(* Logix 5000 AddOnInstructionDefinition export Banner_LE_Param_v4; software revision 33.00 *)

TYPE Banner_IOL_Port_v4 :   // UDT that has all of the data items necessary to communicate with a specific Port on a IO-Link Master
STRUCT
   Port_Controlled : INT;   // Each bit represents a port on an IO-Link Master. Set to 1 to tell AOI to control that port.
   Port_Activate : INT;   // Each bit represents a port on an IO-Link Master. When ON that port will process any commands in queue.
   Port_Read : INT;   // Each bit represents a port on an IO-Link Master. Used to determine when device AOI has requested a Read command.
   Port_Write : INT;   // Each bit represents a port on an IO-Link Master. Used to determine when device AOI has requested a Write command.
   Port_RW_Complete : INT;   // Each bit represents a port on an IO-Link Master. Tells device AOI that Read or Write request has been completed.
   Port_Device_Read : INT;
   Data_Transfer : SINT[190];   // Array to transfer data from IO-Master to device AOIs.
END_STRUCT
END_TYPE

TYPE Banner_LE_RD_v4 :   // UDT with all of the Read only parameters for LE.
STRUCT
   Master_Cycle_Time : INT;
   Min_Cycle_Time : INT;
   M_Sequence_Capability : INT;
   IO_Link_Version_ID : INT;
   Process_Data_Input_Length : INT;
   Process_Data_Output_Length : INT;
   Combined_Vendor_ID : DINT;   // IO-Link Vendor ID
   Vendor_ID1 : INT;
   Vendor_ID2 : INT;
   Combined_Device_ID : DINT;   // IO-Link Device ID
   Device_ID1 : INT;
   Device_ID2 : INT;
   Device_ID3 : INT;
   Serial_Number : STRING;
   Teach_State : SINT;   // 0 =IDLE, 1 = SP1 Success, 4 = Wait for Command, 5 = Busy, 7 = Error
   SP1_TP1 : SINT;   // 0 = not taught or unsuccessful, 1 = successfully taught
   SP2_TP2 : SINT;   // 0 = not taught or unsuccessful, 1 = successfully taught
   Measurement_Value : DINT;   // Measurement value in .1 mm.
   Excess_Gain_Percent : DINT;   // Excess gain expressed as a percentage of minimum signal.
   Stability : INT;   // 0 = No target exists, 1 = Marginal or multiple peaks, 2 = Stable
   Laser_Fault_Status : DINT;   // 0 = No fault, 1 = Laser shut down due to a fault.
   Display_String : STRING;   // String currently being displayed on the LED display of the sensor
END_STRUCT
END_TYPE

TYPE Banner_LE_v4 :   // UDT with all of the parameters for LE.
STRUCT
   Initial_Global_Read : BOOL;   // Determines if all of the IO-Link data has been read into the PLC yet
   Command : INT;   // Value placed in here will activate a read or write to a specifc IO-Link Index
   Read_Data : Banner_LE_RD_v4;   // All read data
   Write_Data : Banner_LE_WD_v4;   // All data that can be written to.
   Archive : Banner_LE_WD_v4;   // Archive of the write data.
   Reset : BOOL;
END_STRUCT
END_TYPE

TYPE Banner_LE_WD_v4 :   // UDT that stores the Write Data for a LE.
STRUCT
   System_Command : INT;   // See IODD file for list of commands that can be activated via the System Command interface
   Parameter_Access_Lock : SINT;   // Write access to all read/write parameters is block when this bit is ON.
   Data_Storage_Lock : SINT;   // Data storage mechanism is inhibited when bit is ON.
   Local_Parameterization_Lock : SINT;   // Parameteriation via local control elementes is inhibited.
   Local_User_Interface_Lock : SINT;   // Operation of the hmi on the device is disabled.
   Teach_Channel : INT;   // 0 = Default, 1 = BDC1, 2 = BDC2
   BDC1_Setpoint_SP1 : DINT;   // SP1 switch point in Switch or Window mode. LE250: Range 100 to 400 (.1 mm increments). LE550: Range 100 to 1000 (.1 mm increments).
   BDC1_Setpoint_SP2 : DINT;   // SP1 switch point in Switch or Window mode. LE250: Range 100 to 400 (.1 mm increments). LE550: Range 100 to 1000 (.1 mm increments).
   BDC1_Swithpoint_Logic : INT;   // Discrete output only. 0 = Light Operate, 1 = Dark Operate
   BDC1_BDC_Mode : INT;   // 1 = Switch Mode/Single Point Mode, 2 = Window Mode, 132 = Health(LO)/Alarm Mode(DO)
   BDC1_Hysteresis : DINT;   // Not Used
   BDC2_Setpoint_SP1 : DINT;   // SP1 switch point in Switch or Window mode. LE250: Range 100 to 400 (.1 mm increments). LE550: Range 100 to 1000 (.1 mm increments).
   BDC2_Setpoint_SP2 : DINT;   // SP1 switch point in Switch or Window mode. LE250: Range 100 to 400 (.1 mm increments). LE550: Range 100 to 1000 (.1 mm increments).
   BDC2_Switchpoint_Logic : INT;   // Discrete output only. 0 = Light Operate, 1 = Dark Operate
   BDC2_BDC_Mode : INT;   // 1 = Switch Mode/Single Point Mode, 2 = Window Mode, 132 = Health(LO)/Alarm Mode(DO)
   BDC2_Hysteresis : DINT;   // Not Used
   Response_Speed : INT;   // 0 = Fast, 1 = Standard, 2 = Medium, 3 = Slow
   Zero_Reference_Location : INT;   // 0 = Near, 1 = Far
   Shift_Zero_Reference_After_Teach : INT;   // 0 = Off, 1 = AutoSet, 2 = SetZero
   Sensor_Lockout : SINT;   // 0 = No Lock Out, 1 = Sensor Locked
   IOL_Filter_Time : DINT;   // Time to average IOL process data measurement between updates. 0 to 65535 ms.
   Display_Read : SINT;   // 0 = Nomral, 1 = Inverted
   Display_Units : SINT;   // 0 = mm, 1 = inches
   Display_Sleep : SINT;   // 0 = 1 min, 1 = 5 min, 2 = 15 min, 3 = 60 min, 4 = Disabled
   Remote_Input_Type : SINT;   // 0 = Teach, 1 = Laser Enable, 2 = Sync Master, 3 = Sync Slave, 4 = Disabled
   BDC1_Delay_Mode : INT;   // 0 = Delay timer disabled, 1 = On & Off Delay, 2 = Off One-Shot timer, 3 = On One-Shot timer
   BDC1_Delay_On_OneShot_Delay : DINT;   // 0 to 9999 ms. 0 ms disables On delay or On/Off oneshot delay.
   BDC1_Delay_Off_OneShot_Delay : DINT;   // 0 to 9999 ms. 0 ms disables Off delay or On/Off oneshot delay.
   BDC1_Switch_Point_Reference : INT;   // 0 = Object, 1 = Background, 2 = Custom
   BDC1_User_Teach_Offset : DINT;   // Range 0 to 32767 (0 to 3276.7 mm)
   BDC1_Midpoint_Window_Size : DINT;   // Range 0 to 32767 (0 to 3276.7 mm)
   BDC1_Midpoint_Teach_Offset_Size : DINT;   // Range 0 to 32767 (0 to 3276.7 mm)
   BDC2_Delay_Mode : INT;   // 0 = Delay timer disabled, 1 = On & Off Delay, 2 = Off One-Shot timer, 3 = On One-Shot timer
   BDC2_Delay_On_OneShot_Delay : DINT;   // 0 to 9999. 0 ms disables On delay or On/Off oneshot delay.
   BDC2_Delay_Off_OneShot_Delay : DINT;   // 0 to 9999. 0 ms disables Off delay or On/Off oneshot delay.
   BDC2_Switch_Point_Reference : INT;   // 0 = Object, 1 = Background, 2 = Custom
   BDC2_User_Teach_Offset : DINT;   // Range 0 to 32767 (0 to 3276.7 mm)
   BDC2_Midpoint_Window_Size : DINT;   // Range 0 to 32767 (0 to 3276.7 mm)
   BDC2_Midpoint_Teach_Offset_Size : DINT;   // Range 0 to 32767 (0 to 3276.7 mm)
END_STRUCT
END_TYPE

ADD_ON_INSTRUCTION Banner_LE_Param_v4   (* revision 4.0, vendor Banner Engineering *)
// AOI to read and write parameter data to an IO-Link LE.
VAR_IN_OUT
   LE : Banner_LE_v4; {required}
   Port_Data : Banner_IOL_Port_v4; {required}
END_VAR
VAR_INPUT
   Port : DINT; {required}
END_VAR
VAR
   Local_Control : DINT; {access None}
   Global_Read_Command_Value : INT; {access None}
   Global_Write_Command_Value : INT; {access None}
   Command_Being_Processed : BOOL; {access None}
   Update_Archive : BOOL; {access None}
   Index_Write_Control : DINT; {access None}
   Index_Write_Inprocess : INT; {access None}
   Temp_Excess_Gain : DINT[2]; {access None}
   Inprocess_Index : DINT; {access None}
END_VAR

ROUTINE Logic   (* ladder *)
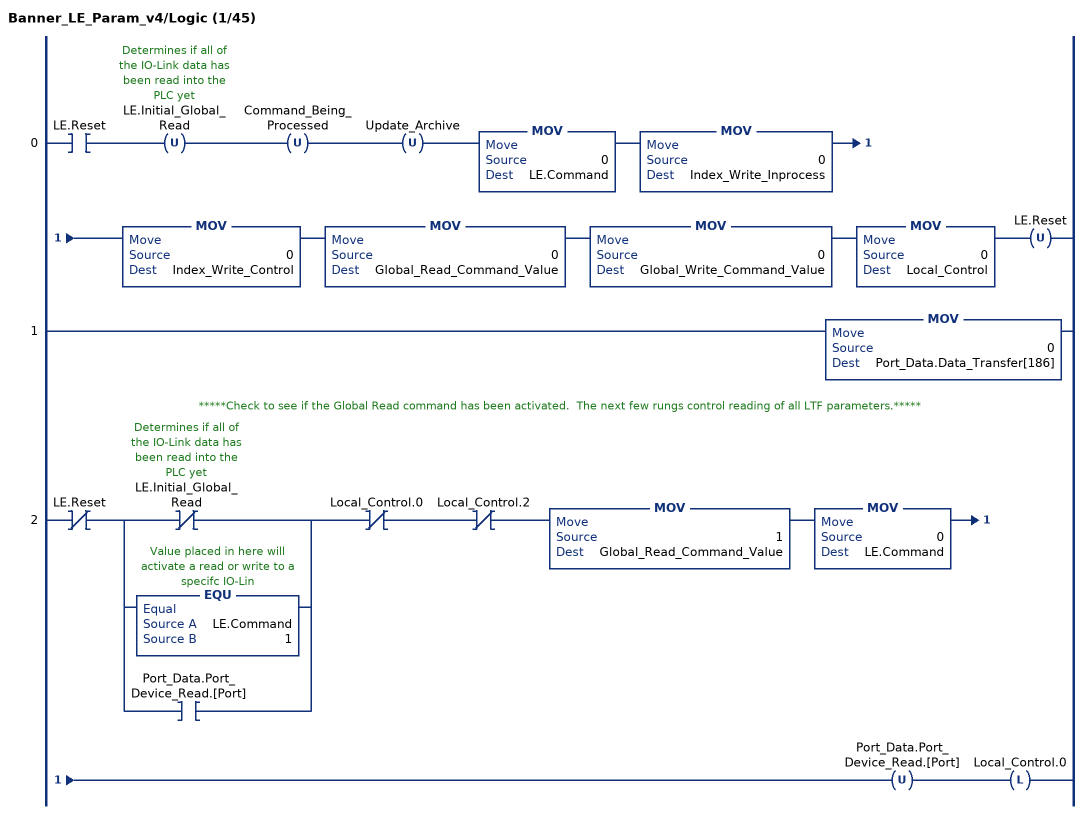
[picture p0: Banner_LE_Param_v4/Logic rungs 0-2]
   0: XIC(LE.Reset)OTU(LE.Initial_Global_Read)OTU(Command_Being_Processed)OTU(Update_Archive)MOV(0,LE.Command)MOV(0,Index_Write_Inprocess)MOV(0,Index_Write_Control)MOV(0,Global_Read_Command_Value)MOV(0,Global_Write_Command_Value)MOV(0,Local_Control)OTU(LE.Reset);
   1: MOV(0,Port_Data.Data_Transfer[186]);
   // *****Check to see if the Global Read command has been activated.  The next few rungs control reading of all LTF parameters.*****
   2: XIO(LE.Reset)[XIO(LE.Initial_Global_Read) ,EQU(LE.Command,1) ,XIC(Port_Data.Port_Device_Read.[Port]) ]XIO(Local_Control.0)XIO(Local_Control.2)MOV(1,Global_Read_Command_Value)MOV(0,LE.Command)OTU(Port_Data.Port_Device_Read.[Port])OTL(Local_Control.0);
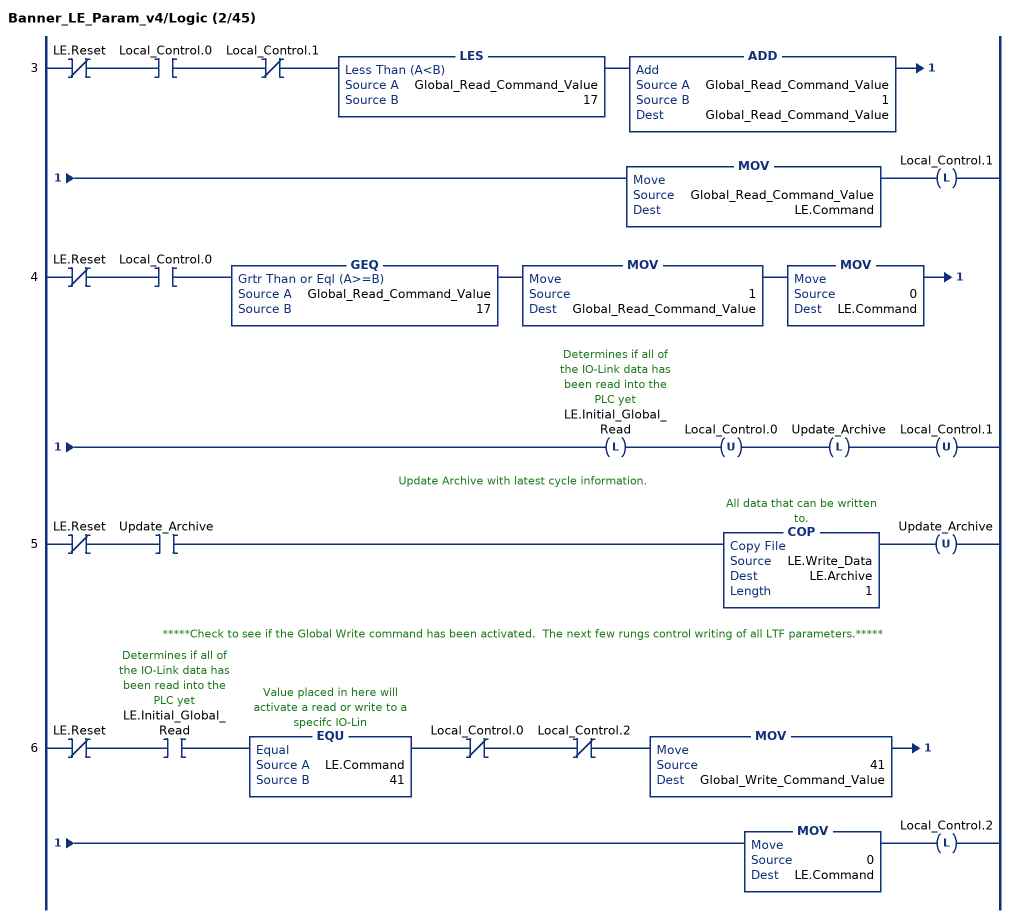
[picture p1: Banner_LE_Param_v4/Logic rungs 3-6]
   3: XIO(LE.Reset)XIC(Local_Control.0)XIO(Local_Control.1)LES(Global_Read_Command_Value,17)ADD(Global_Read_Command_Value,1,Global_Read_Command_Value)MOV(Global_Read_Command_Value,LE.Command)OTL(Local_Control.1);
   4: XIO(LE.Reset)XIC(Local_Control.0)GEQ(Global_Read_Command_Value,17)MOV(1,Global_Read_Command_Value)MOV(0,LE.Command)OTL(LE.Initial_Global_Read)OTU(Local_Control.0)OTL(Update_Archive)OTU(Local_Control.1);
   // Update Archive with latest cycle information.
   5: XIO(LE.Reset)XIC(Update_Archive)COP(LE.Write_Data,LE.Archive,1)OTU(Update_Archive);
   // *****Check to see if the Global Write command has been activated.  The next few rungs control writing of all LTF parameters.*****
   6: XIO(LE.Reset)XIC(LE.Initial_Global_Read)EQU(LE.Command,41)XIO(Local_Control.0)XIO(Local_Control.2)MOV(41,Global_Write_Command_Value)MOV(0,LE.Command)OTL(Local_Control.2);
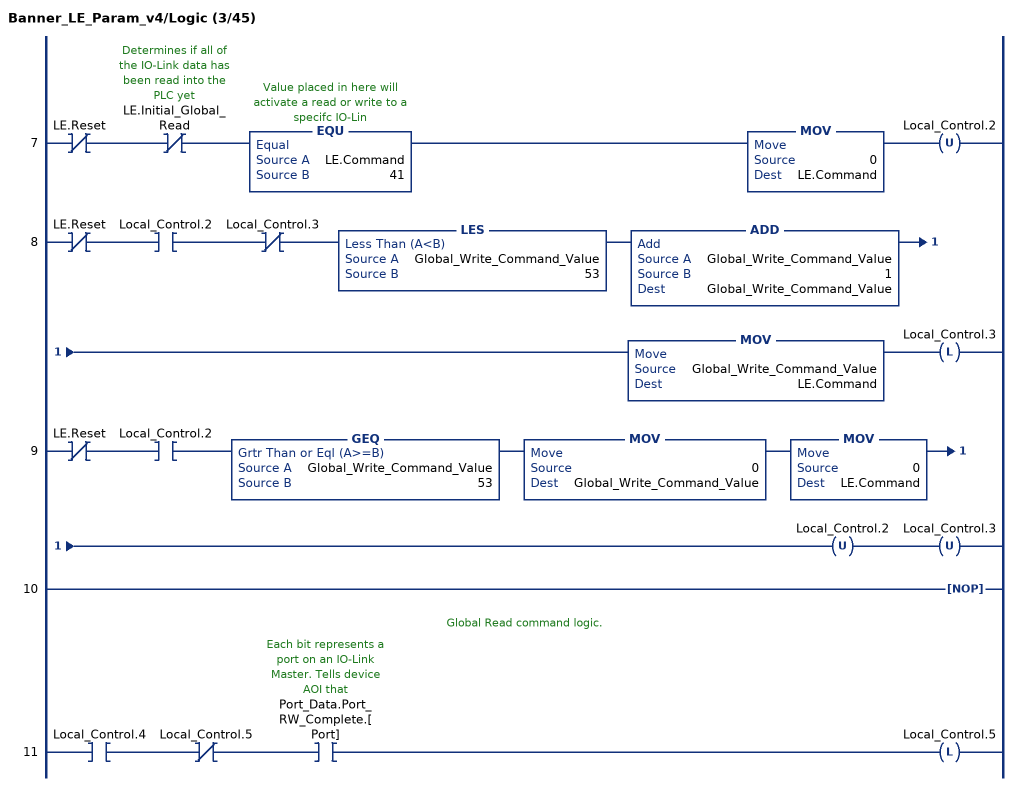
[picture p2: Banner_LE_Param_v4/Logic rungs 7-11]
   7: XIO(LE.Reset)XIO(LE.Initial_Global_Read)EQU(LE.Command,41)MOV(0,LE.Command)OTU(Local_Control.2);
   8: XIO(LE.Reset)XIC(Local_Control.2)XIO(Local_Control.3)LES(Global_Write_Command_Value,53)ADD(Global_Write_Command_Value,1,Global_Write_Command_Value)MOV(Global_Write_Command_Value,LE.Command)OTL(Local_Control.3);
   9: XIO(LE.Reset)XIC(Local_Control.2)GEQ(Global_Write_Command_Value,53)MOV(0,Global_Write_Command_Value)MOV(0,LE.Command)OTU(Local_Control.2)OTU(Local_Control.3);
   10: NOP();
   // Global Read command logic.
   11: XIC(Local_Control.4)XIO(Local_Control.5)XIC(Port_Data.Port_RW_Complete.[Port])OTL(Local_Control.5);
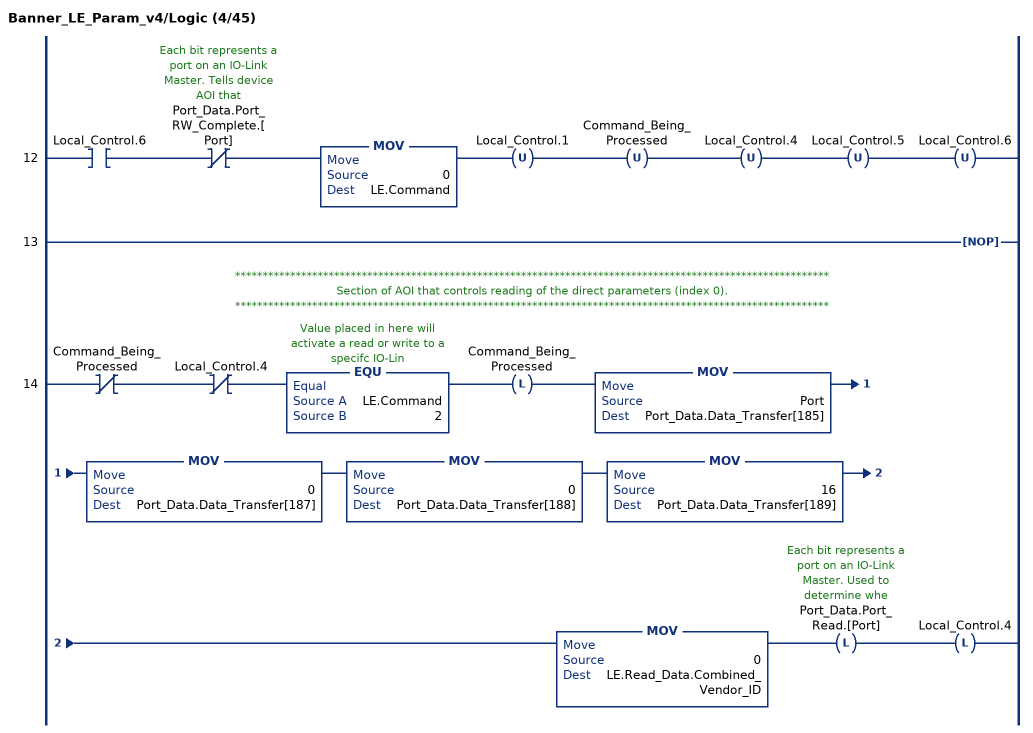
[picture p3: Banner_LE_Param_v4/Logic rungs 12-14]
   12: XIC(Local_Control.6)XIO(Port_Data.Port_RW_Complete.[Port])MOV(0,LE.Command)OTU(Local_Control.1)OTU(Command_Being_Processed)OTU(Local_Control.4)OTU(Local_Control.5)OTU(Local_Control.6);
   13: NOP();
   // ************************************************************************************************************
   // Section of AOI that controls reading of the direct parameters (index 0).
   // ************************************************************************************************************
   14: XIO(Command_Being_Processed)XIO(Local_Control.4)EQU(LE.Command,2)OTL(Command_Being_Processed)MOV(Port,Port_Data.Data_Transfer[185])MOV(0,Port_Data.Data_Transfer[187])MOV(0,Port_Data.Data_Transfer[188])MOV(16,Port_Data.Data_Transfer[189])MOV(0,LE.Read_Data.Combined_Vendor_ID)OTL(Port_Data.Port_Read.[Port])OTL(Local_Control.4);
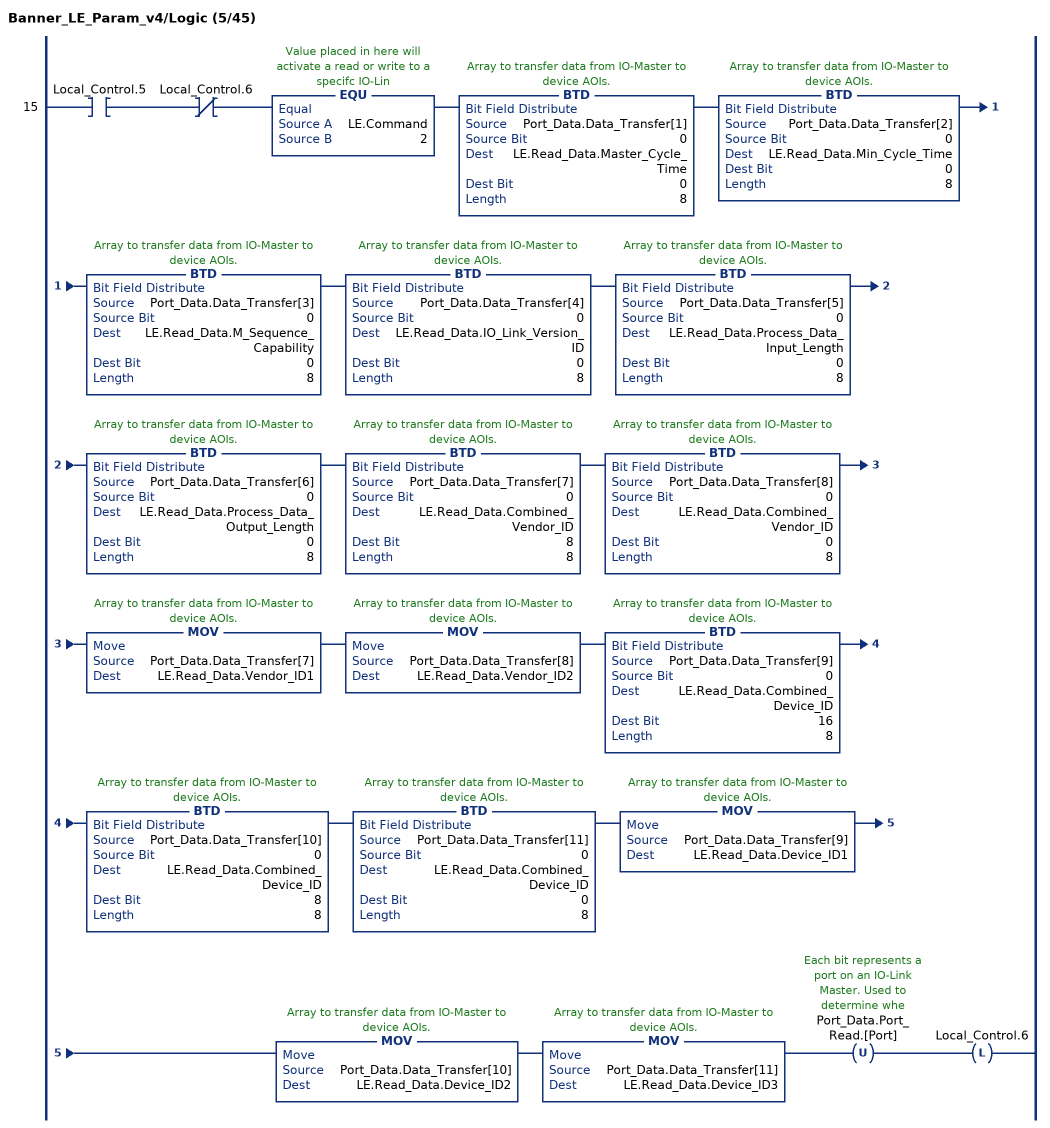
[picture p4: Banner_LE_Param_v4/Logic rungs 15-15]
   15: XIC(Local_Control.5)XIO(Local_Control.6)EQU(LE.Command,2)BTD(Port_Data.Data_Transfer[1],0,LE.Read_Data.Master_Cycle_Time,0,8)BTD(Port_Data.Data_Transfer[2],0,LE.Read_Data.Min_Cycle_Time,0,8)BTD(Port_Data.Data_Transfer[3],0,LE.Read_Data.M_Sequence_Capability,0,8)BTD(Port_Data.Data_Transfer[4],0,LE.Read_Data.IO_Link_Version_ID,0,8)BTD(Port_Data.Data_Transfer[5],0,LE.Read_Data.Process_Data_Input_Length,0,8)BTD(Port_Data.Data_Transfer[6],0,LE.Read_Data.Process_Data_Output_Length,0,8)BTD(Port_Data.Data_Transfer[7],0,LE.Read_Data.Combined_Vendor_ID,8,8)BTD(Port_Data.Data_Transfer[8],0,LE.Read_Data.Combined_Vendor_ID,0,8)MOV(Port_Data.Data_Transfer[7],LE.Read_Data.Vendor_ID1)MOV(Port_Data.Data_Transfer[8],LE.Read_Data.Vendor_ID2)BTD(Port_Data.Data_Transfer[9],0,LE.Read_Data.Combined_Device_ID,16,8)BTD(Port_Data.Data_Transfer[10],0,LE.Read_Data.Combined_Device_ID,8,8)BTD(Port_Data.Data_Transfer[11],0,LE.Read_Data.Combined_Device_ID,0,8)MOV(Port_Data.Data_Transfer[9],LE.Read_Data.Device_ID1)MOV(Port_Data.Data_Transfer[10],LE.Read_Data.Device_ID2)MOV(Port_Data.Data_Transfer[11],LE.Read_Data.Device_ID3)OTU(Port_Data.Port_Read.[Port])OTL(Local_Control.6);
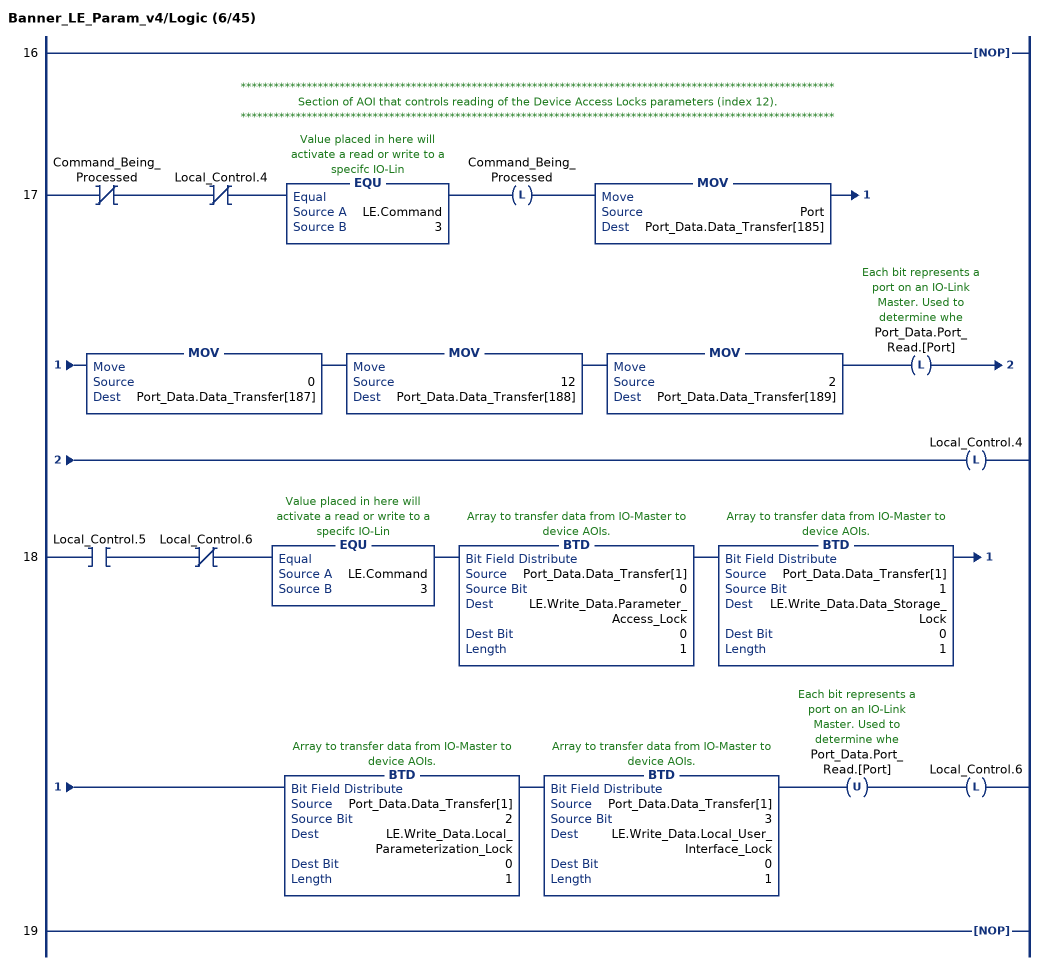
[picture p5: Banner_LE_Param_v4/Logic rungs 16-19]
   16: NOP();
   // ************************************************************************************************************
   // Section of AOI that controls reading of the Device Access Locks parameters (index 12).
   // ************************************************************************************************************
   17: XIO(Command_Being_Processed)XIO(Local_Control.4)EQU(LE.Command,3)OTL(Command_Being_Processed)MOV(Port,Port_Data.Data_Transfer[185])MOV(0,Port_Data.Data_Transfer[187])MOV(12,Port_Data.Data_Transfer[188])MOV(2,Port_Data.Data_Transfer[189])OTL(Port_Data.Port_Read.[Port])OTL(Local_Control.4);
   18: XIC(Local_Control.5)XIO(Local_Control.6)EQU(LE.Command,3)BTD(Port_Data.Data_Transfer[1],0,LE.Write_Data.Parameter_Access_Lock,0,1)BTD(Port_Data.Data_Transfer[1],1,LE.Write_Data.Data_Storage_Lock,0,1)BTD(Port_Data.Data_Transfer[1],2,LE.Write_Data.Local_Parameterization_Lock,0,1)BTD(Port_Data.Data_Transfer[1],3,LE.Write_Data.Local_User_Interface_Lock,0,1)OTU(Port_Data.Port_Read.[Port])OTL(Local_Control.6);
   19: NOP();
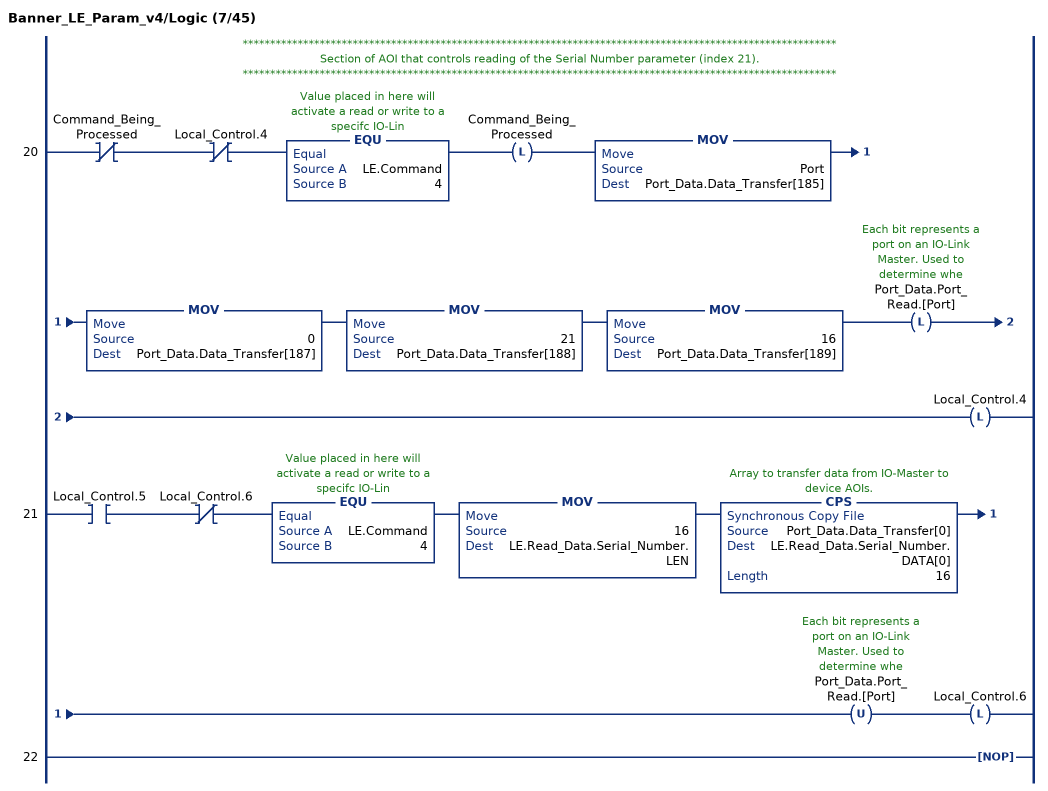
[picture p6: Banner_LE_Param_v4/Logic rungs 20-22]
   // ************************************************************************************************************
   // Section of AOI that controls reading of the Serial Number parameter (index 21).
   // ************************************************************************************************************
   20: XIO(Command_Being_Processed)XIO(Local_Control.4)EQU(LE.Command,4)OTL(Command_Being_Processed)MOV(Port,Port_Data.Data_Transfer[185])MOV(0,Port_Data.Data_Transfer[187])MOV(21,Port_Data.Data_Transfer[188])MOV(16,Port_Data.Data_Transfer[189])OTL(Port_Data.Port_Read.[Port])OTL(Local_Control.4);
   21: XIC(Local_Control.5)XIO(Local_Control.6)EQU(LE.Command,4)MOV(16,LE.Read_Data.Serial_Number.LEN)CPS(Port_Data.Data_Transfer[0],LE.Read_Data.Serial_Number.DATA[0],16)OTU(Port_Data.Port_Read.[Port])OTL(Local_Control.6);
   22: NOP();
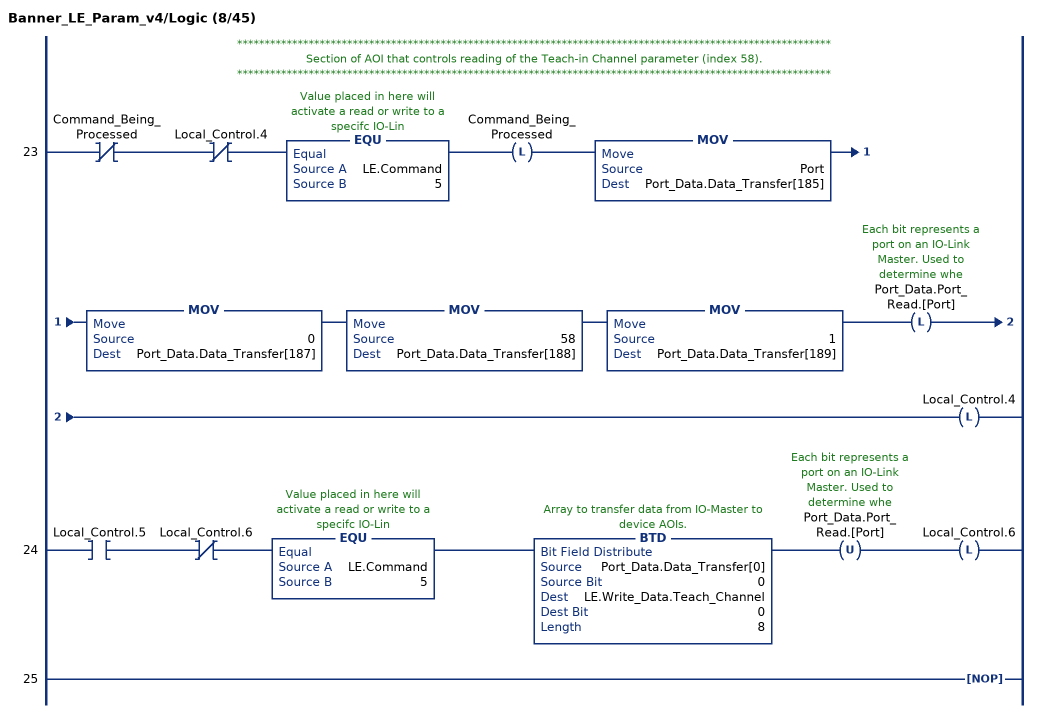
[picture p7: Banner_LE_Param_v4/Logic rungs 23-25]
   // ************************************************************************************************************
   // Section of AOI that controls reading of the Teach-in Channel parameter (index 58).
   // ************************************************************************************************************
   23: XIO(Command_Being_Processed)XIO(Local_Control.4)EQU(LE.Command,5)OTL(Command_Being_Processed)MOV(Port,Port_Data.Data_Transfer[185])MOV(0,Port_Data.Data_Transfer[187])MOV(58,Port_Data.Data_Transfer[188])MOV(1,Port_Data.Data_Transfer[189])OTL(Port_Data.Port_Read.[Port])OTL(Local_Control.4);
   24: XIC(Local_Control.5)XIO(Local_Control.6)EQU(LE.Command,5)BTD(Port_Data.Data_Transfer[0],0,LE.Write_Data.Teach_Channel,0,8)OTU(Port_Data.Port_Read.[Port])OTL(Local_Control.6);
   25: NOP();
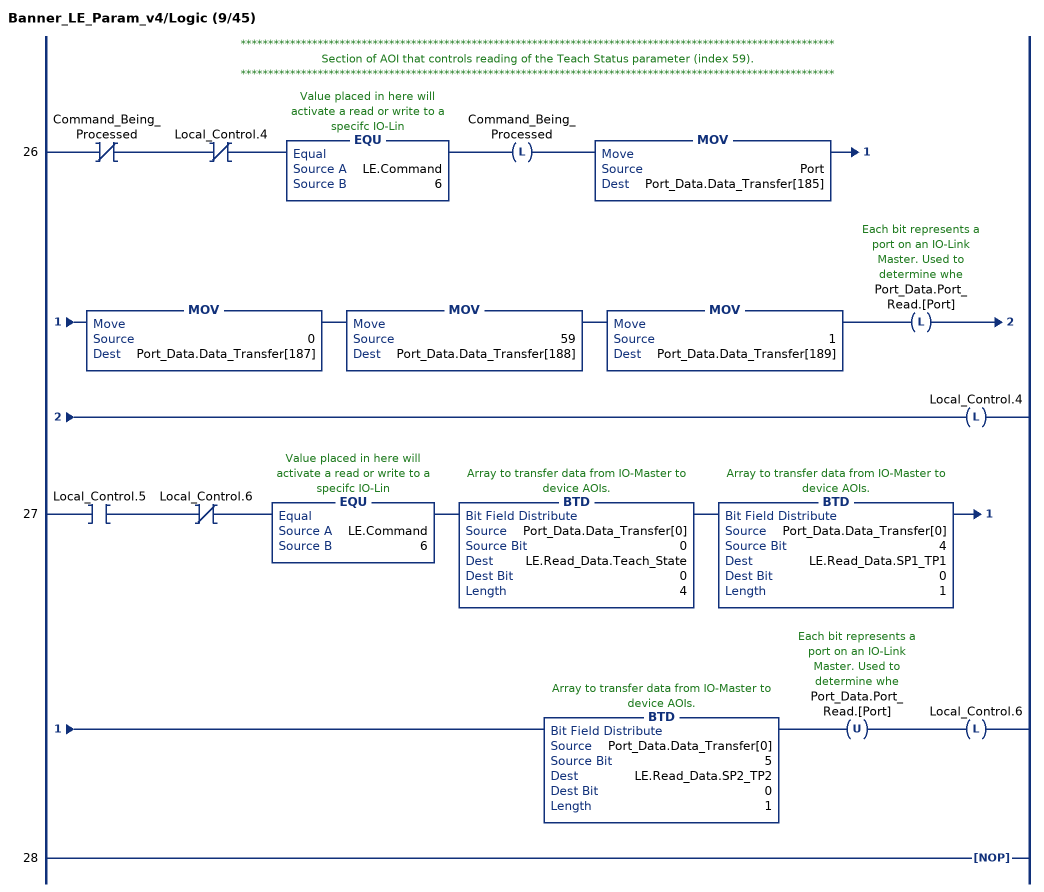
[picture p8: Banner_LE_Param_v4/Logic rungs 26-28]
   // ************************************************************************************************************
   // Section of AOI that controls reading of the Teach Status parameter (index 59).
   // ************************************************************************************************************
   26: XIO(Command_Being_Processed)XIO(Local_Control.4)EQU(LE.Command,6)OTL(Command_Being_Processed)MOV(Port,Port_Data.Data_Transfer[185])MOV(0,Port_Data.Data_Transfer[187])MOV(59,Port_Data.Data_Transfer[188])MOV(1,Port_Data.Data_Transfer[189])OTL(Port_Data.Port_Read.[Port])OTL(Local_Control.4);
   27: XIC(Local_Control.5)XIO(Local_Control.6)EQU(LE.Command,6)BTD(Port_Data.Data_Transfer[0],0,LE.Read_Data.Teach_State,0,4)BTD(Port_Data.Data_Transfer[0],4,LE.Read_Data.SP1_TP1,0,1)BTD(Port_Data.Data_Transfer[0],5,LE.Read_Data.SP2_TP2,0,1)OTU(Port_Data.Port_Read.[Port])OTL(Local_Control.6);
   28: NOP();
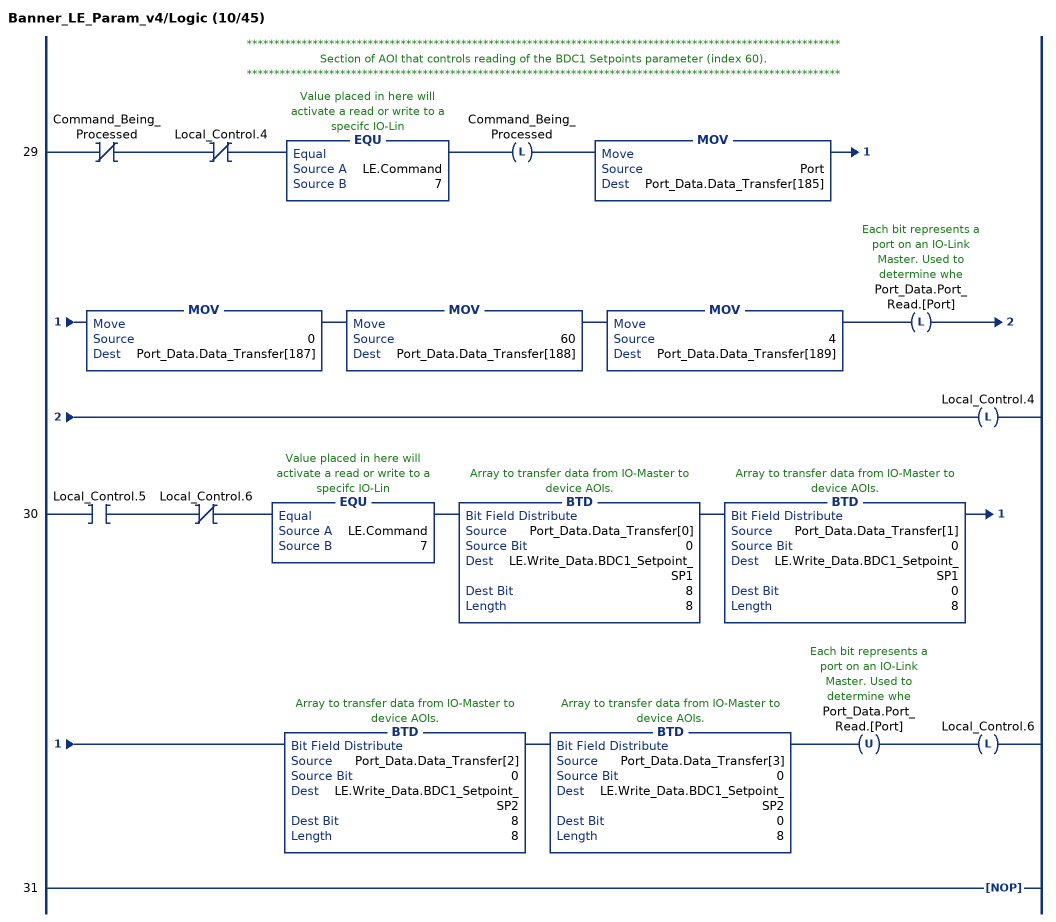
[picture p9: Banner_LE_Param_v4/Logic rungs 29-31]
   // ************************************************************************************************************
   // Section of AOI that controls reading of the BDC1 Setpoints parameter (index 60).
   // ************************************************************************************************************
   29: XIO(Command_Being_Processed)XIO(Local_Control.4)EQU(LE.Command,7)OTL(Command_Being_Processed)MOV(Port,Port_Data.Data_Transfer[185])MOV(0,Port_Data.Data_Transfer[187])MOV(60,Port_Data.Data_Transfer[188])MOV(4,Port_Data.Data_Transfer[189])OTL(Port_Data.Port_Read.[Port])OTL(Local_Control.4);
   30: XIC(Local_Control.5)XIO(Local_Control.6)EQU(LE.Command,7)BTD(Port_Data.Data_Transfer[0],0,LE.Write_Data.BDC1_Setpoint_SP1,8,8)BTD(Port_Data.Data_Transfer[1],0,LE.Write_Data.BDC1_Setpoint_SP1,0,8)BTD(Port_Data.Data_Transfer[2],0,LE.Write_Data.BDC1_Setpoint_SP2,8,8)BTD(Port_Data.Data_Transfer[3],0,LE.Write_Data.BDC1_Setpoint_SP2,0,8)OTU(Port_Data.Port_Read.[Port])OTL(Local_Control.6);
   31: NOP();
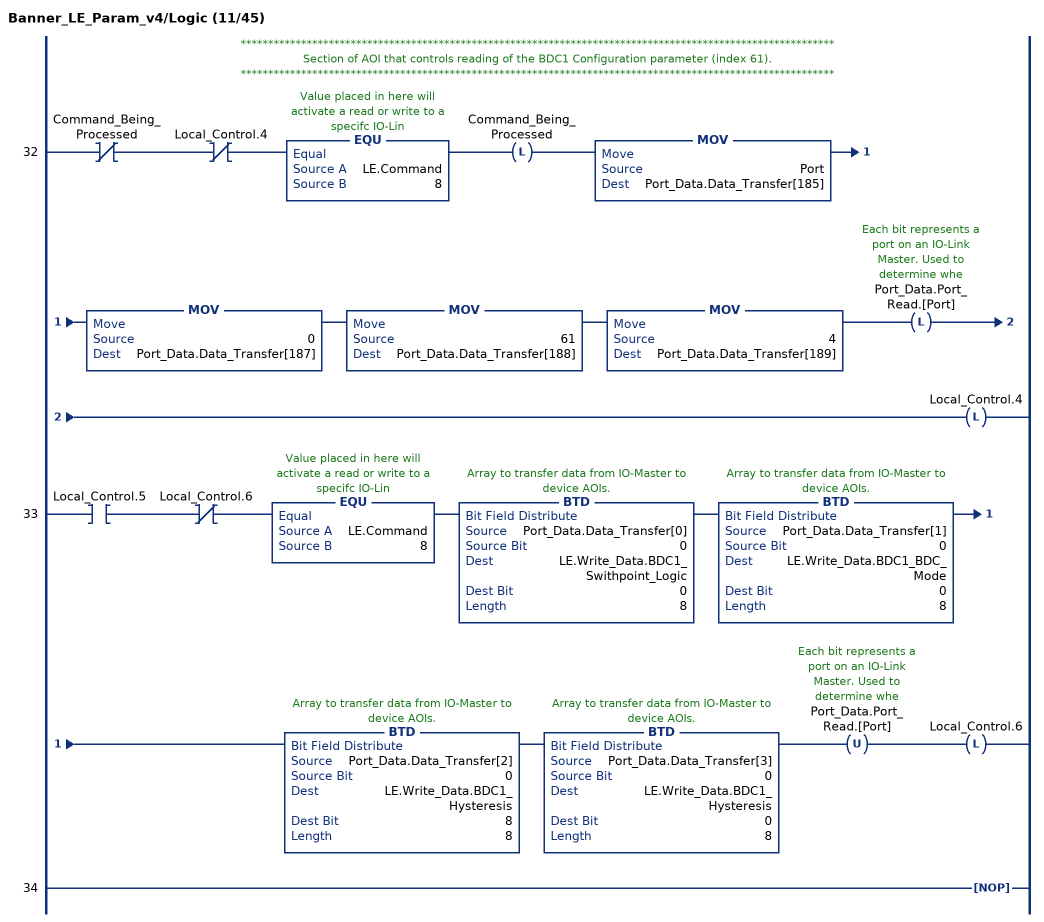
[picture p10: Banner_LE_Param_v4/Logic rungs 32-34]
   // ************************************************************************************************************
   // Section of AOI that controls reading of the BDC1 Configuration parameter (index 61).
   // ************************************************************************************************************
   32: XIO(Command_Being_Processed)XIO(Local_Control.4)EQU(LE.Command,8)OTL(Command_Being_Processed)MOV(Port,Port_Data.Data_Transfer[185])MOV(0,Port_Data.Data_Transfer[187])MOV(61,Port_Data.Data_Transfer[188])MOV(4,Port_Data.Data_Transfer[189])OTL(Port_Data.Port_Read.[Port])OTL(Local_Control.4);
   33: XIC(Local_Control.5)XIO(Local_Control.6)EQU(LE.Command,8)BTD(Port_Data.Data_Transfer[0],0,LE.Write_Data.BDC1_Swithpoint_Logic,0,8)BTD(Port_Data.Data_Transfer[1],0,LE.Write_Data.BDC1_BDC_Mode,0,8)BTD(Port_Data.Data_Transfer[2],0,LE.Write_Data.BDC1_Hysteresis,8,8)BTD(Port_Data.Data_Transfer[3],0,LE.Write_Data.BDC1_Hysteresis,0,8)OTU(Port_Data.Port_Read.[Port])OTL(Local_Control.6);
   34: NOP();
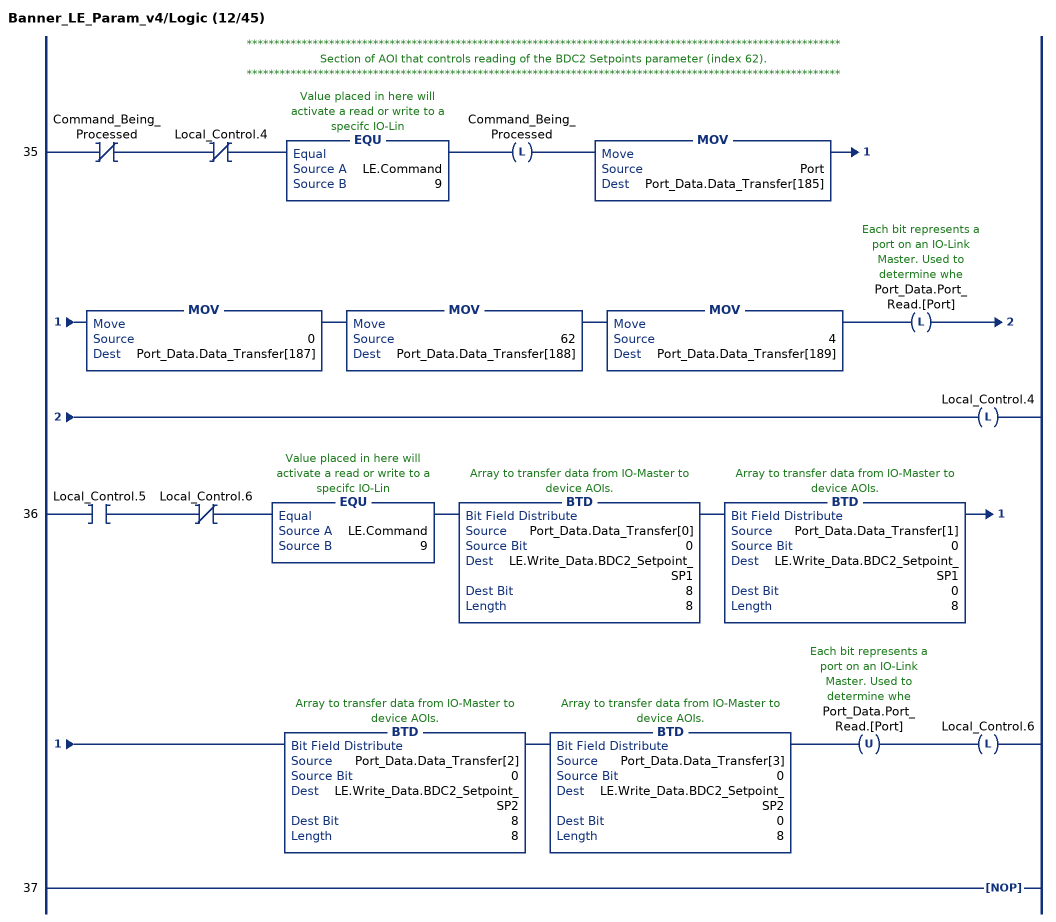
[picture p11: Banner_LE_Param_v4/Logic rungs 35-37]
   // ************************************************************************************************************
   // Section of AOI that controls reading of the BDC2 Setpoints parameter (index 62).
   // ************************************************************************************************************
   35: XIO(Command_Being_Processed)XIO(Local_Control.4)EQU(LE.Command,9)OTL(Command_Being_Processed)MOV(Port,Port_Data.Data_Transfer[185])MOV(0,Port_Data.Data_Transfer[187])MOV(62,Port_Data.Data_Transfer[188])MOV(4,Port_Data.Data_Transfer[189])OTL(Port_Data.Port_Read.[Port])OTL(Local_Control.4);
   36: XIC(Local_Control.5)XIO(Local_Control.6)EQU(LE.Command,9)BTD(Port_Data.Data_Transfer[0],0,LE.Write_Data.BDC2_Setpoint_SP1,8,8)BTD(Port_Data.Data_Transfer[1],0,LE.Write_Data.BDC2_Setpoint_SP1,0,8)BTD(Port_Data.Data_Transfer[2],0,LE.Write_Data.BDC2_Setpoint_SP2,8,8)BTD(Port_Data.Data_Transfer[3],0,LE.Write_Data.BDC2_Setpoint_SP2,0,8)OTU(Port_Data.Port_Read.[Port])OTL(Local_Control.6);
   37: NOP();
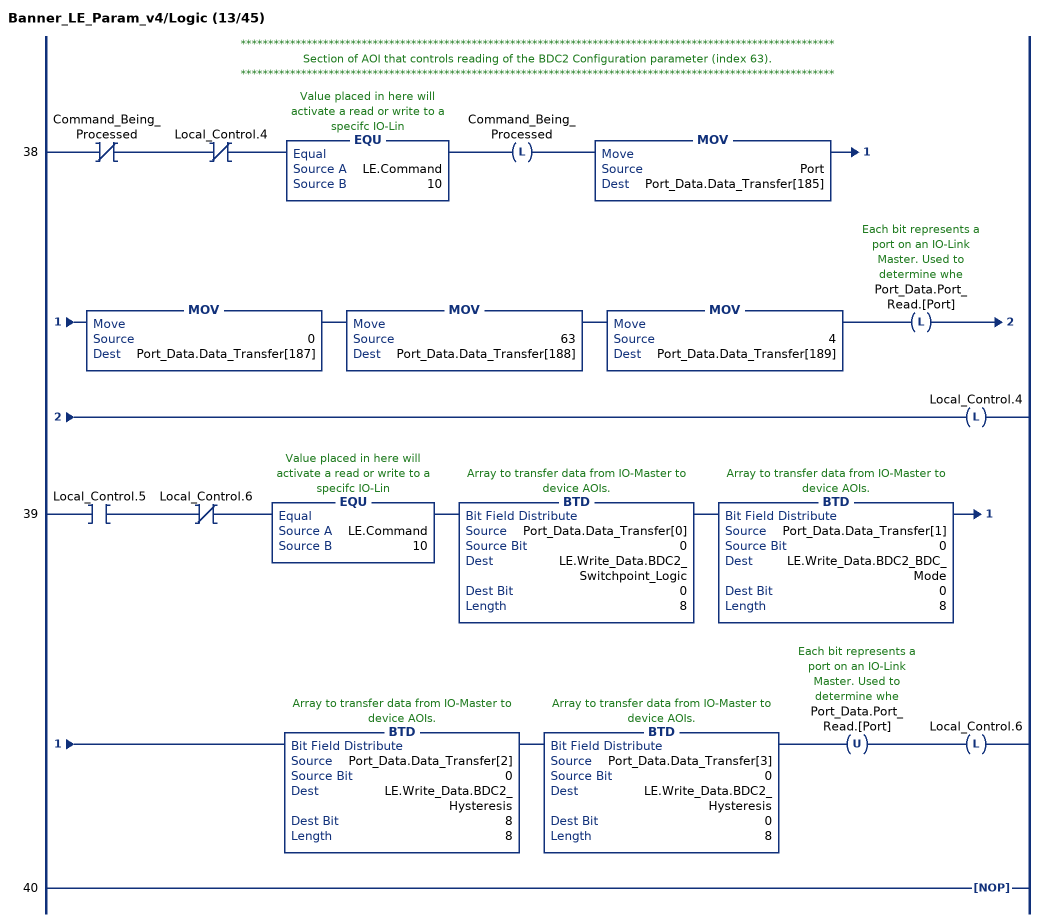
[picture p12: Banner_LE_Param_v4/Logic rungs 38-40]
   // ************************************************************************************************************
   // Section of AOI that controls reading of the BDC2 Configuration parameter (index 63).
   // ************************************************************************************************************
   38: XIO(Command_Being_Processed)XIO(Local_Control.4)EQU(LE.Command,10)OTL(Command_Being_Processed)MOV(Port,Port_Data.Data_Transfer[185])MOV(0,Port_Data.Data_Transfer[187])MOV(63,Port_Data.Data_Transfer[188])MOV(4,Port_Data.Data_Transfer[189])OTL(Port_Data.Port_Read.[Port])OTL(Local_Control.4);
   39: XIC(Local_Control.5)XIO(Local_Control.6)EQU(LE.Command,10)BTD(Port_Data.Data_Transfer[0],0,LE.Write_Data.BDC2_Switchpoint_Logic,0,8)BTD(Port_Data.Data_Transfer[1],0,LE.Write_Data.BDC2_BDC_Mode,0,8)BTD(Port_Data.Data_Transfer[2],0,LE.Write_Data.BDC2_Hysteresis,8,8)BTD(Port_Data.Data_Transfer[3],0,LE.Write_Data.BDC2_Hysteresis,0,8)OTU(Port_Data.Port_Read.[Port])OTL(Local_Control.6);
   40: NOP();
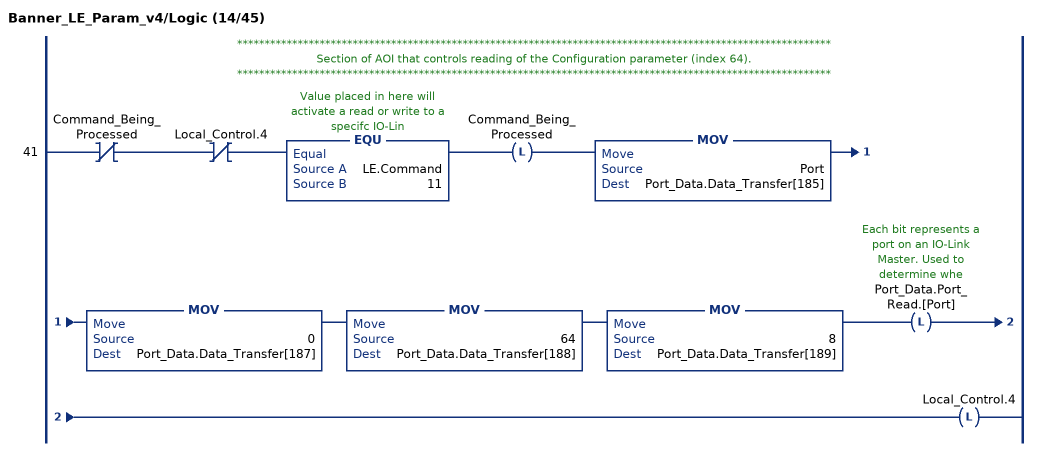
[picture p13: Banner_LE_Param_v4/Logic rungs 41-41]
   // ************************************************************************************************************
   // Section of AOI that controls reading of the Configuration parameter (index 64).
   // ************************************************************************************************************
   41: XIO(Command_Being_Processed)XIO(Local_Control.4)EQU(LE.Command,11)OTL(Command_Being_Processed)MOV(Port,Port_Data.Data_Transfer[185])MOV(0,Port_Data.Data_Transfer[187])MOV(64,Port_Data.Data_Transfer[188])MOV(8,Port_Data.Data_Transfer[189])OTL(Port_Data.Port_Read.[Port])OTL(Local_Control.4);
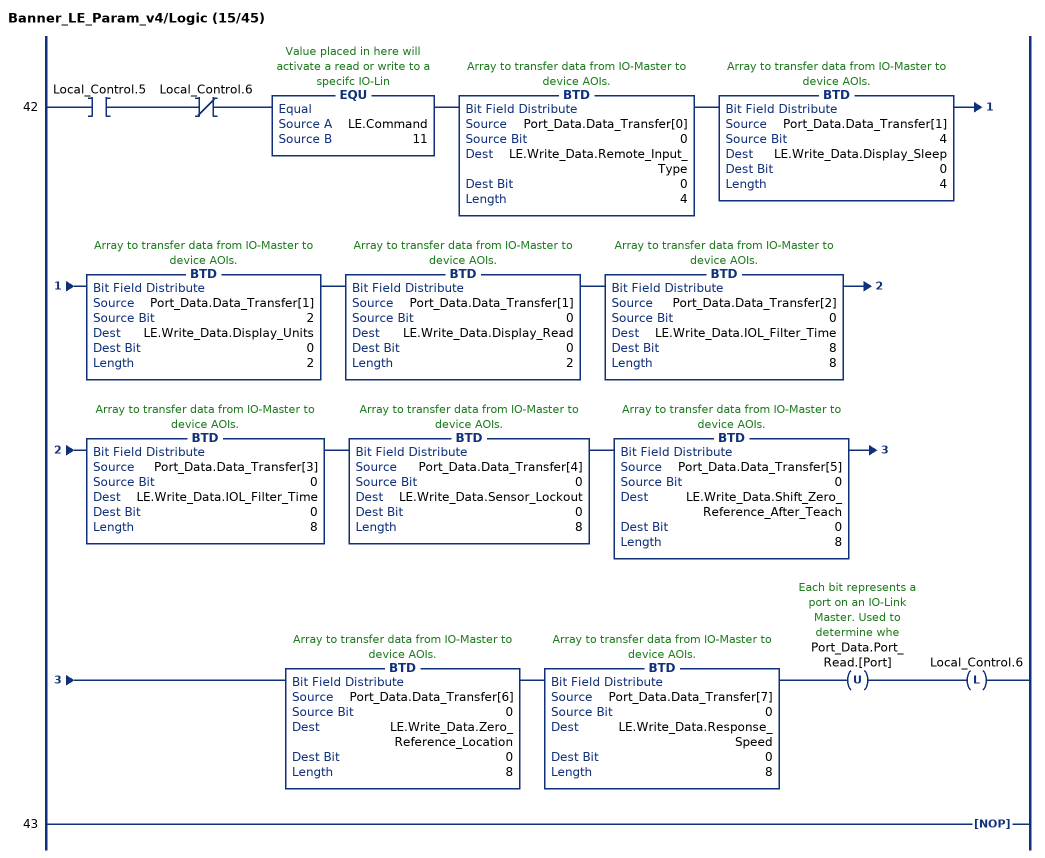
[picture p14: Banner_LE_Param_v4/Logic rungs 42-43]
   42: XIC(Local_Control.5)XIO(Local_Control.6)EQU(LE.Command,11)BTD(Port_Data.Data_Transfer[0],0,LE.Write_Data.Remote_Input_Type,0,4)BTD(Port_Data.Data_Transfer[1],4,LE.Write_Data.Display_Sleep,0,4)BTD(Port_Data.Data_Transfer[1],2,LE.Write_Data.Display_Units,0,2)BTD(Port_Data.Data_Transfer[1],0,LE.Write_Data.Display_Read,0,2)BTD(Port_Data.Data_Transfer[2],0,LE.Write_Data.IOL_Filter_Time,8,8)BTD(Port_Data.Data_Transfer[3],0,LE.Write_Data.IOL_Filter_Time,0,8)BTD(Port_Data.Data_Transfer[4],0,LE.Write_Data.Sensor_Lockout,0,8)BTD(Port_Data.Data_Transfer[5],0,LE.Write_Data.Shift_Zero_Reference_After_Teach,0,8)BTD(Port_Data.Data_Transfer[6],0,LE.Write_Data.Zero_Reference_Location,0,8)BTD(Port_Data.Data_Transfer[7],0,LE.Write_Data.Response_Speed,0,8)OTU(Port_Data.Port_Read.[Port])OTL(Local_Control.6);
   43: NOP();
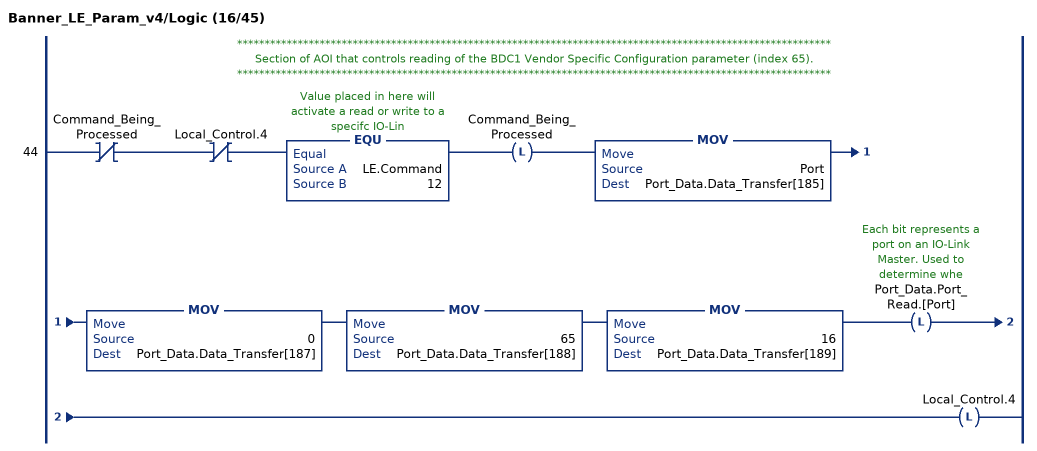
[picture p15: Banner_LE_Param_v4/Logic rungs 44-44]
   // ************************************************************************************************************
   // Section of AOI that controls reading of the BDC1 Vendor Specific Configuration parameter (index 65).
   // ************************************************************************************************************
   44: XIO(Command_Being_Processed)XIO(Local_Control.4)EQU(LE.Command,12)OTL(Command_Being_Processed)MOV(Port,Port_Data.Data_Transfer[185])MOV(0,Port_Data.Data_Transfer[187])MOV(65,Port_Data.Data_Transfer[188])MOV(16,Port_Data.Data_Transfer[189])OTL(Port_Data.Port_Read.[Port])OTL(Local_Control.4);
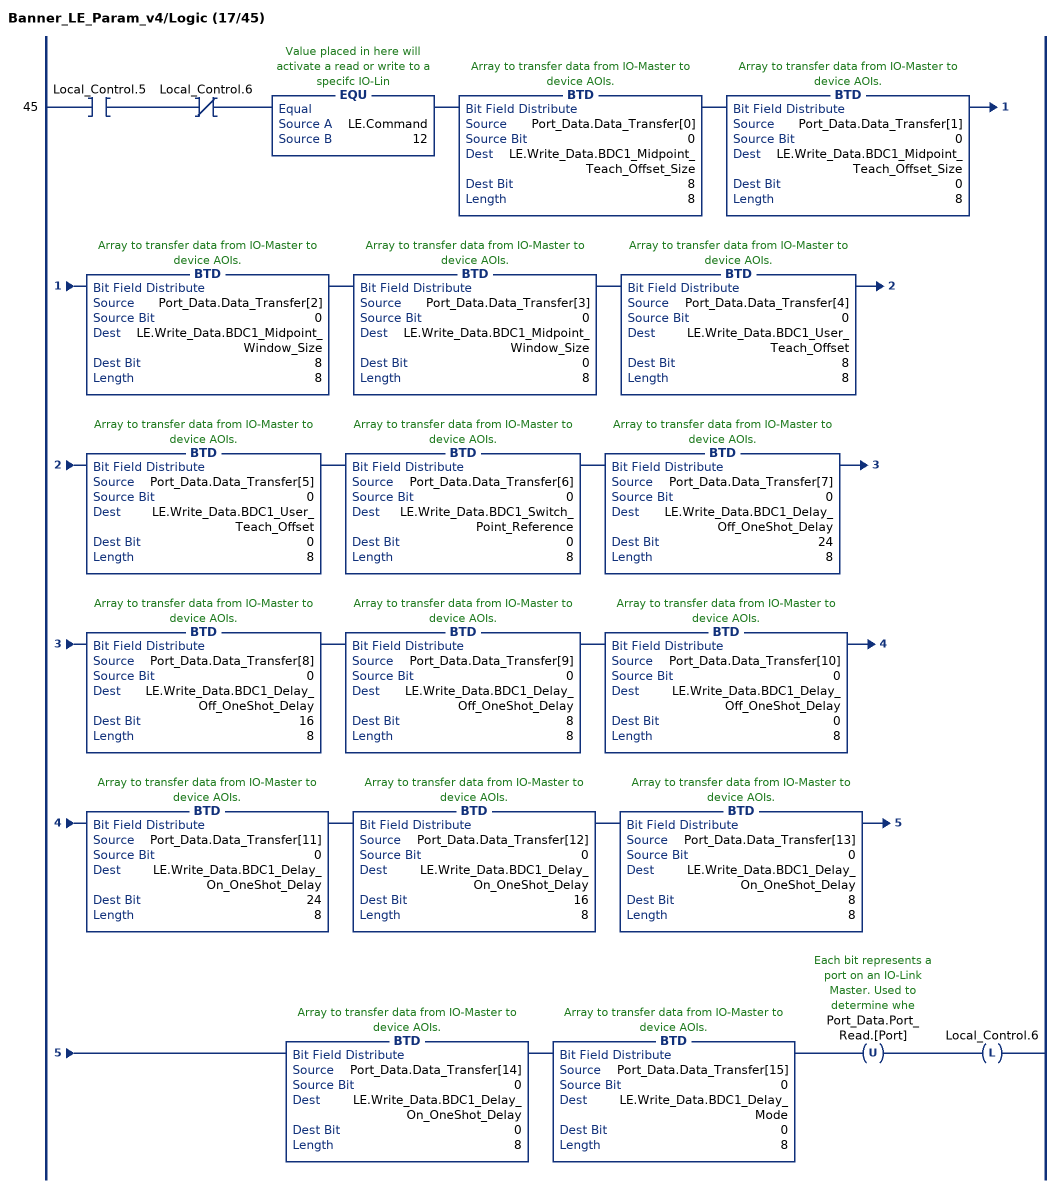
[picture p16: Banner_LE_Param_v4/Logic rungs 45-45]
   45: XIC(Local_Control.5)XIO(Local_Control.6)EQU(LE.Command,12)BTD(Port_Data.Data_Transfer[0],0,LE.Write_Data.BDC1_Midpoint_Teach_Offset_Size,8,8)BTD(Port_Data.Data_Transfer[1],0,LE.Write_Data.BDC1_Midpoint_Teach_Offset_Size,0,8)BTD(Port_Data.Data_Transfer[2],0,LE.Write_Data.BDC1_Midpoint_Window_Size,8,8)BTD(Port_Data.Data_Transfer[3],0,LE.Write_Data.BDC1_Midpoint_Window_Size,0,8)BTD(Port_Data.Data_Transfer[4],0,LE.Write_Data.BDC1_User_Teach_Offset,8,8)BTD(Port_Data.Data_Transfer[5],0,LE.Write_Data.BDC1_User_Teach_Offset,0,8)BTD(Port_Data.Data_Transfer[6],0,LE.Write_Data.BDC1_Switch_Point_Reference,0,8)BTD(Port_Data.Data_Transfer[7],0,LE.Write_Data.BDC1_Delay_Off_OneShot_Delay,24,8)BTD(Port_Data.Data_Transfer[8],0,LE.Write_Data.BDC1_Delay_Off_OneShot_Delay,16,8)BTD(Port_Data.Data_Transfer[9],0,LE.Write_Data.BDC1_Delay_Off_OneShot_Delay,8,8)BTD(Port_Data.Data_Transfer[10],0,LE.Write_Data.BDC1_Delay_Off_OneShot_Delay,0,8)BTD(Port_Data.Data_Transfer[11],0,LE.Write_Data.BDC1_Delay_On_OneShot_Delay,24,8)BTD(Port_Data.Data_Transfer[12],0,LE.Write_Data.BDC1_Delay_On_OneShot_Delay,16,8)BTD(Port_Data.Data_Transfer[13],0,LE.Write_Data.BDC1_Delay_On_OneShot_Delay,8,8)BTD(Port_Data.Data_Transfer[14],0,LE.Write_Data.BDC1_Delay_On_OneShot_Delay,0,8)BTD(Port_Data.Data_Transfer[15],0,LE.Write_Data.BDC1_Delay_Mode,0,8)OTU(Port_Data.Port_Read.[Port])OTL(Local_Control.6);
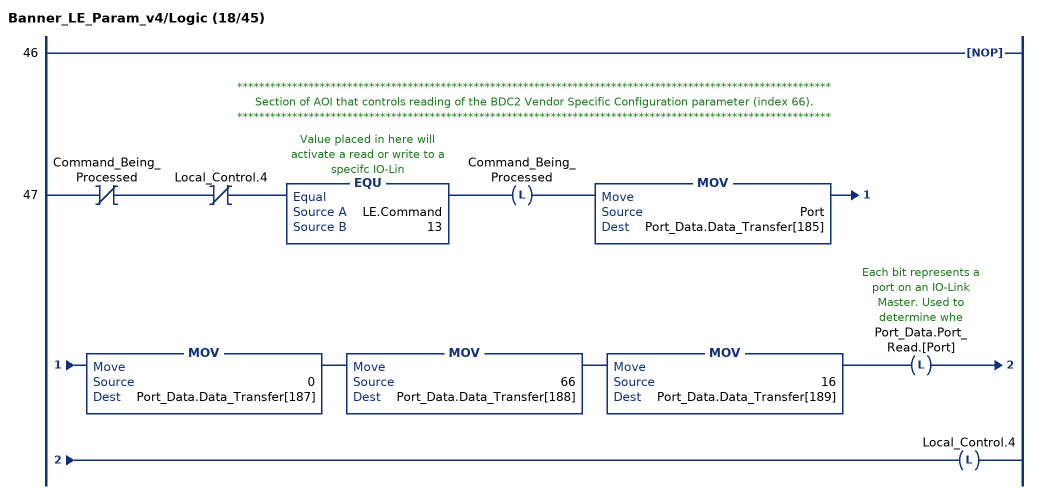
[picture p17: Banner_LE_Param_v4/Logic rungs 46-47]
   46: NOP();
   // ************************************************************************************************************
   // Section of AOI that controls reading of the BDC2 Vendor Specific Configuration parameter (index 66).
   // ************************************************************************************************************
   47: XIO(Command_Being_Processed)XIO(Local_Control.4)EQU(LE.Command,13)OTL(Command_Being_Processed)MOV(Port,Port_Data.Data_Transfer[185])MOV(0,Port_Data.Data_Transfer[187])MOV(66,Port_Data.Data_Transfer[188])MOV(16,Port_Data.Data_Transfer[189])OTL(Port_Data.Port_Read.[Port])OTL(Local_Control.4);
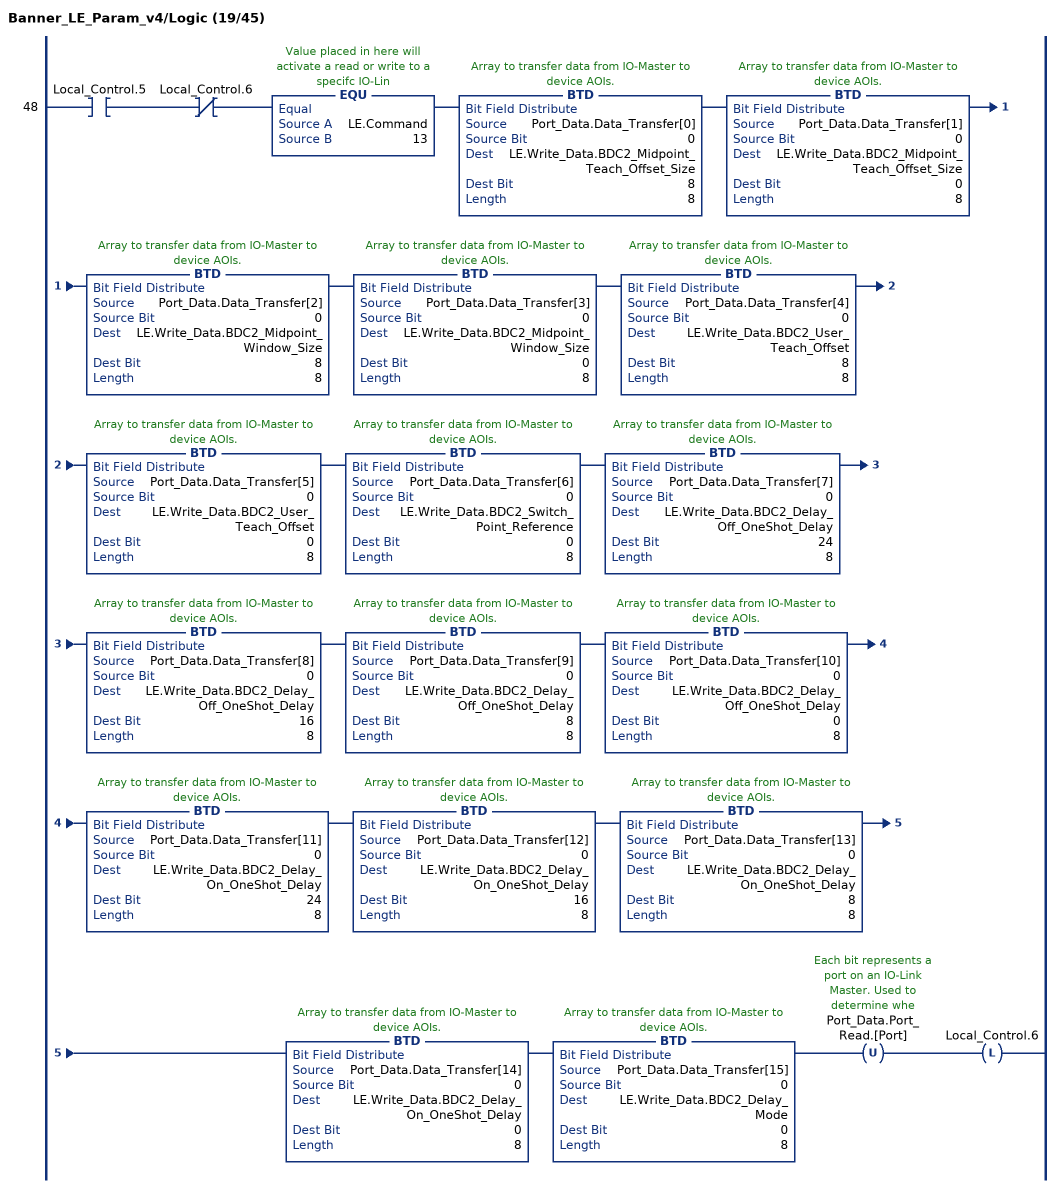
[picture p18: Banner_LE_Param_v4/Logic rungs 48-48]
   48: XIC(Local_Control.5)XIO(Local_Control.6)EQU(LE.Command,13)BTD(Port_Data.Data_Transfer[0],0,LE.Write_Data.BDC2_Midpoint_Teach_Offset_Size,8,8)BTD(Port_Data.Data_Transfer[1],0,LE.Write_Data.BDC2_Midpoint_Teach_Offset_Size,0,8)BTD(Port_Data.Data_Transfer[2],0,LE.Write_Data.BDC2_Midpoint_Window_Size,8,8)BTD(Port_Data.Data_Transfer[3],0,LE.Write_Data.BDC2_Midpoint_Window_Size,0,8)BTD(Port_Data.Data_Transfer[4],0,LE.Write_Data.BDC2_User_Teach_Offset,8,8)BTD(Port_Data.Data_Transfer[5],0,LE.Write_Data.BDC2_User_Teach_Offset,0,8)BTD(Port_Data.Data_Transfer[6],0,LE.Write_Data.BDC2_Switch_Point_Reference,0,8)BTD(Port_Data.Data_Transfer[7],0,LE.Write_Data.BDC2_Delay_Off_OneShot_Delay,24,8)BTD(Port_Data.Data_Transfer[8],0,LE.Write_Data.BDC2_Delay_Off_OneShot_Delay,16,8)BTD(Port_Data.Data_Transfer[9],0,LE.Write_Data.BDC2_Delay_Off_OneShot_Delay,8,8)BTD(Port_Data.Data_Transfer[10],0,LE.Write_Data.BDC2_Delay_Off_OneShot_Delay,0,8)BTD(Port_Data.Data_Transfer[11],0,LE.Write_Data.BDC2_Delay_On_OneShot_Delay,24,8)BTD(Port_Data.Data_Transfer[12],0,LE.Write_Data.BDC2_Delay_On_OneShot_Delay,16,8)BTD(Port_Data.Data_Transfer[13],0,LE.Write_Data.BDC2_Delay_On_OneShot_Delay,8,8)BTD(Port_Data.Data_Transfer[14],0,LE.Write_Data.BDC2_Delay_On_OneShot_Delay,0,8)BTD(Port_Data.Data_Transfer[15],0,LE.Write_Data.BDC2_Delay_Mode,0,8)OTU(Port_Data.Port_Read.[Port])OTL(Local_Control.6);
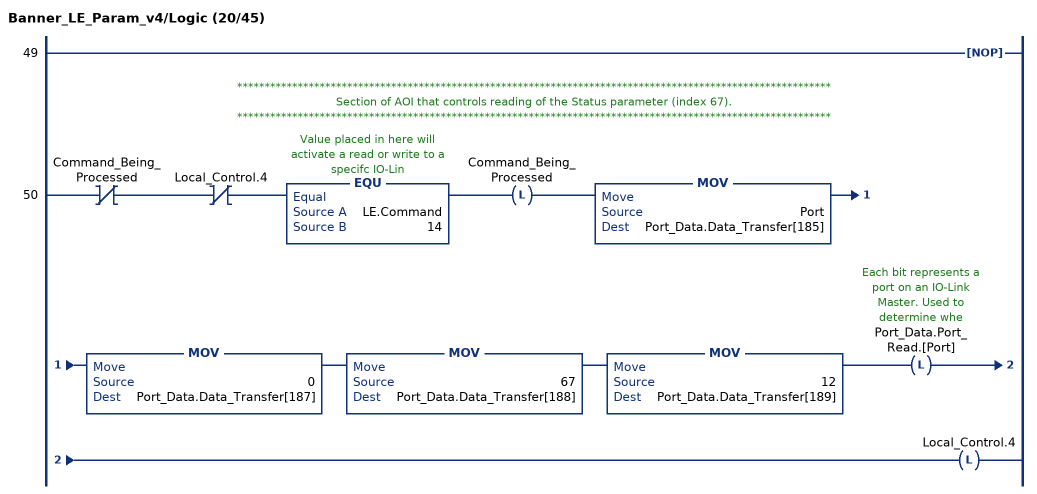
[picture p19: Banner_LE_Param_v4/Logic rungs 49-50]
   49: NOP();
   // ************************************************************************************************************
   // Section of AOI that controls reading of the Status parameter (index 67).
   // ************************************************************************************************************
   50: XIO(Command_Being_Processed)XIO(Local_Control.4)EQU(LE.Command,14)OTL(Command_Being_Processed)MOV(Port,Port_Data.Data_Transfer[185])MOV(0,Port_Data.Data_Transfer[187])MOV(67,Port_Data.Data_Transfer[188])MOV(12,Port_Data.Data_Transfer[189])OTL(Port_Data.Port_Read.[Port])OTL(Local_Control.4);
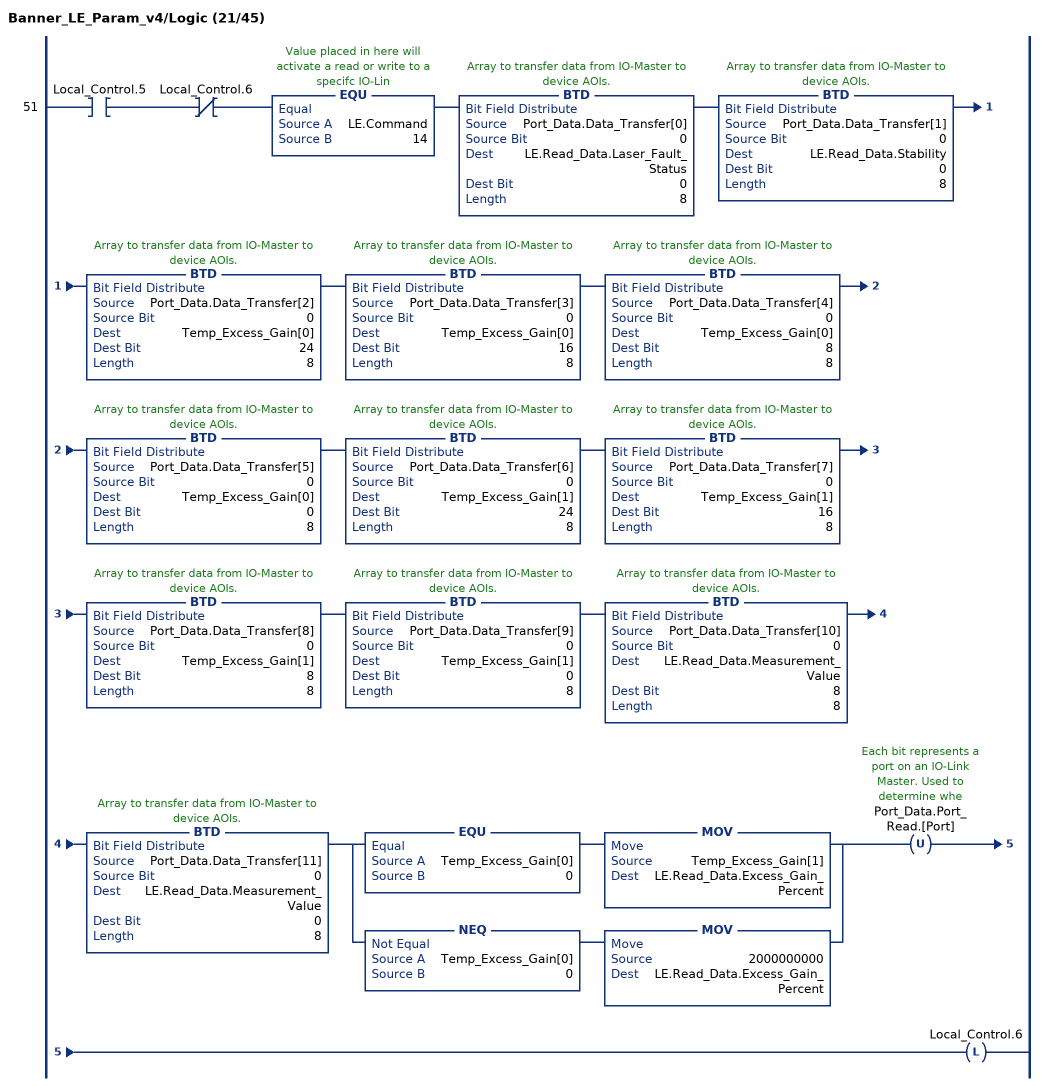
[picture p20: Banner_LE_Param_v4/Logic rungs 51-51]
   51: XIC(Local_Control.5)XIO(Local_Control.6)EQU(LE.Command,14)BTD(Port_Data.Data_Transfer[0],0,LE.Read_Data.Laser_Fault_Status,0,8)BTD(Port_Data.Data_Transfer[1],0,LE.Read_Data.Stability,0,8)BTD(Port_Data.Data_Transfer[2],0,Temp_Excess_Gain[0],24,8)BTD(Port_Data.Data_Transfer[3],0,Temp_Excess_Gain[0],16,8)BTD(Port_Data.Data_Transfer[4],0,Temp_Excess_Gain[0],8,8)BTD(Port_Data.Data_Transfer[5],0,Temp_Excess_Gain[0],0,8)BTD(Port_Data.Data_Transfer[6],0,Temp_Excess_Gain[1],24,8)BTD(Port_Data.Data_Transfer[7],0,Temp_Excess_Gain[1],16,8)BTD(Port_Data.Data_Transfer[8],0,Temp_Excess_Gain[1],8,8)BTD(Port_Data.Data_Transfer[9],0,Temp_Excess_Gain[1],0,8)BTD(Port_Data.Data_Transfer[10],0,LE.Read_Data.Measurement_Value,8,8)BTD(Port_Data.Data_Transfer[11],0,LE.Read_Data.Measurement_Value,0,8)[EQU(Temp_Excess_Gain[0],0) MOV(Temp_Excess_Gain[1],LE.Read_Data.Excess_Gain_Percent) ,NEQ(Temp_Excess_Gain[0],0) MOV(2000000000,LE.Read_Data.Excess_Gain_Percent) ]OTU(Port_Data.Port_Read.[Port])OTL(Local_Control.6);
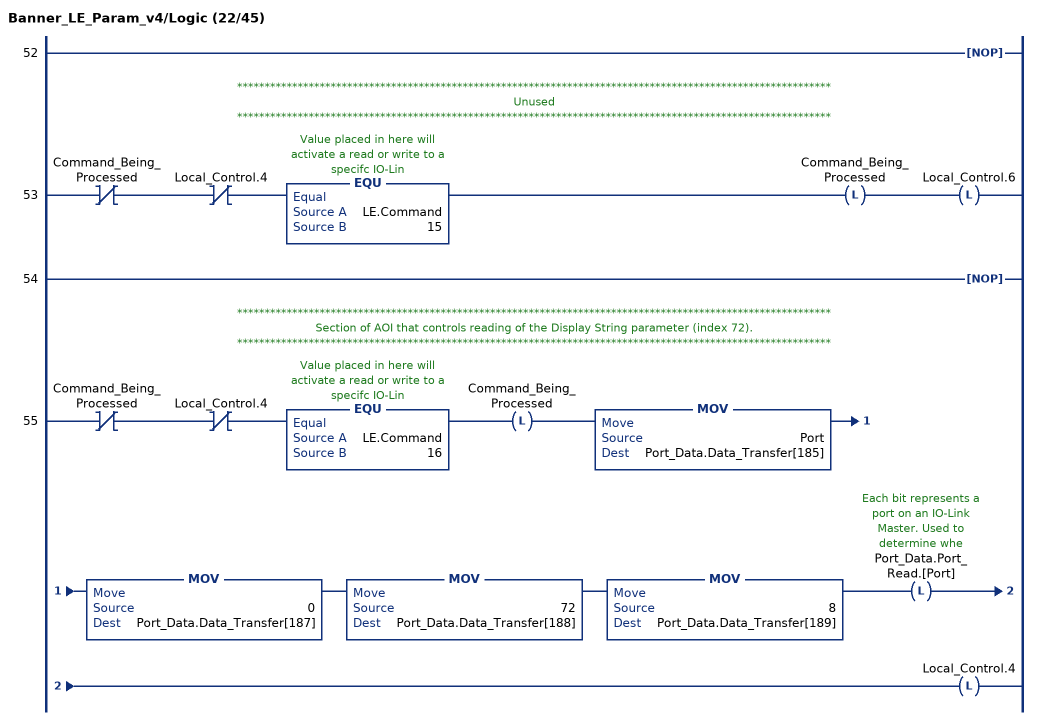
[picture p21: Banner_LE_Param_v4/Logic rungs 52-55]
   52: NOP();
   // ************************************************************************************************************
   // Unused
   // ************************************************************************************************************
   53: XIO(Command_Being_Processed)XIO(Local_Control.4)EQU(LE.Command,15)OTL(Command_Being_Processed)OTL(Local_Control.6);
   54: NOP();
   // ************************************************************************************************************
   // Section of AOI that controls reading of the Display String parameter (index 72).
   // ************************************************************************************************************
   55: XIO(Command_Being_Processed)XIO(Local_Control.4)EQU(LE.Command,16)OTL(Command_Being_Processed)MOV(Port,Port_Data.Data_Transfer[185])MOV(0,Port_Data.Data_Transfer[187])MOV(72,Port_Data.Data_Transfer[188])MOV(8,Port_Data.Data_Transfer[189])OTL(Port_Data.Port_Read.[Port])OTL(Local_Control.4);
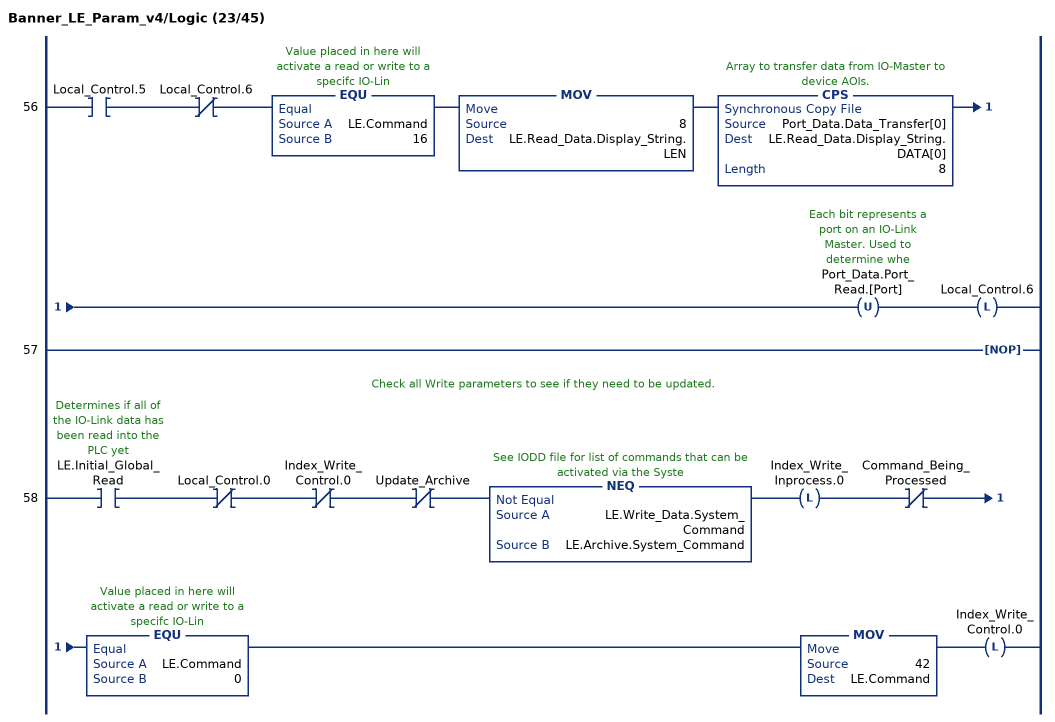
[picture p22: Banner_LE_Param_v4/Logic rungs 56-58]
   56: XIC(Local_Control.5)XIO(Local_Control.6)EQU(LE.Command,16)MOV(8,LE.Read_Data.Display_String.LEN)CPS(Port_Data.Data_Transfer[0],LE.Read_Data.Display_String.DATA[0],8)OTU(Port_Data.Port_Read.[Port])OTL(Local_Control.6);
   57: NOP();
   // Check all Write parameters to see if they need to be updated.
   58: XIC(LE.Initial_Global_Read)XIO(Local_Control.0)XIO(Index_Write_Control.0)XIO(Update_Archive)NEQ(LE.Write_Data.System_Command,LE.Archive.System_Command)OTL(Index_Write_Inprocess.0)XIO(Command_Being_Processed)EQU(LE.Command,0)MOV(42,LE.Command)OTL(Index_Write_Control.0);
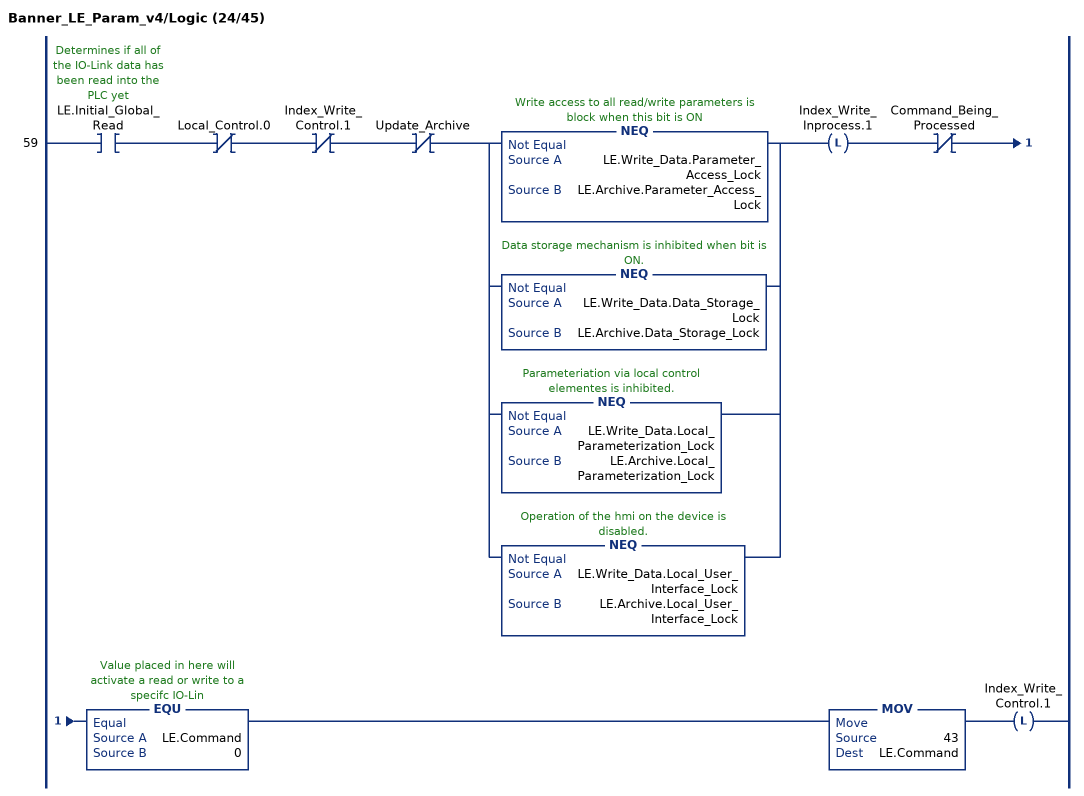
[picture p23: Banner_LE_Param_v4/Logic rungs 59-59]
   59: XIC(LE.Initial_Global_Read)XIO(Local_Control.0)XIO(Index_Write_Control.1)XIO(Update_Archive)[NEQ(LE.Write_Data.Parameter_Access_Lock,LE.Archive.Parameter_Access_Lock) ,NEQ(LE.Write_Data.Data_Storage_Lock,LE.Archive.Data_Storage_Lock) ,NEQ(LE.Write_Data.Local_Parameterization_Lock,LE.Archive.Local_Parameterization_Lock) ,NEQ(LE.Write_Data.Local_User_Interface_Lock,LE.Archive.Local_User_Interface_Lock) ]OTL(Index_Write_Inprocess.1)XIO(Command_Being_Processed)EQU(LE.Command,0)MOV(43,LE.Command)OTL(Index_Write_Control.1);
